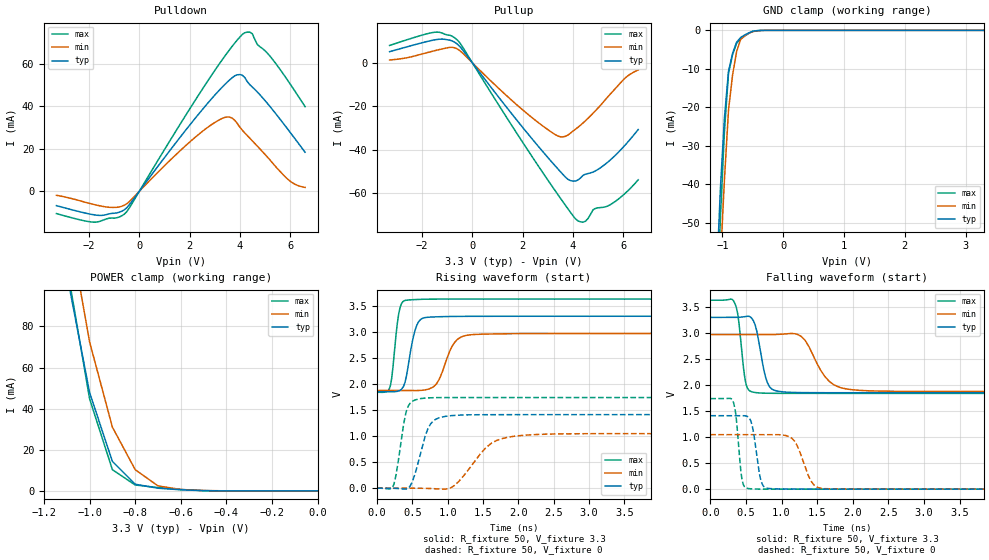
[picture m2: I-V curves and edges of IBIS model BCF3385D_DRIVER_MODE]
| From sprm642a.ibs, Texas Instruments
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|   Model Cell BCF3385D_DRIVER_MODE
|BCF3385D_DRIVER_MODE
[Model]   BCF3385D_DRIVER_MODE
Model_type   I/O
Polarity   Non-Inverting
Enable   Active-Low
Vinl =  0.8
Vinh =  2
Cref =  15.0000pF
Rref =  100.0000M
Vref =  0V
Vmeas =  1.65
C_comp   1.187844p   1.059102p   1.312744p
[Model Spec]
Vinl   0.8   0.8   0.8
Vinh   2   2   2
[Temperature Range]   25   155   -40
[Voltage Range]   3.3   2.97   3.63
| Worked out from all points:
|   slope of the pulldown table from 0 to 0.495 V, typ, clamps not added: 62.6 ohm
|   slope of the pullup table from 0 to 0.495 V, typ, clamps not added: 65.4 ohm
|   GND clamp passes 1 mA (typ) near -0.61 V on its own axis
|   POWER clamp passes 1 mA (typ) near -0.66 V on its own axis
|   rising waveform, R_fixture 50, V_fixture 3.3: 20-80 % time 120ps typ, 194ps min, 83.7ps max; typ from 1.85 V to 3.3 V
|   rising waveform, R_fixture 50, V_fixture 0: 20-80 % time 178ps typ, 387ps min, 119ps max; typ from 0 V to 1.41 V
|   falling waveform, R_fixture 50, V_fixture 3.3: 20-80 % time 122ps typ, 275ps min, 84ps max; typ from 3.3 V to 1.85 V
|   falling waveform, R_fixture 50, V_fixture 0: 20-80 % time 90.6ps typ, 176ps min, 67.2ps max; typ from 1.41 V to 0 V
| Nom Voltages:
|   VDD=1.2, VDDS=3.3, VSS=0
| Min Voltages:
|   VDD=1.08, VDDS=2.97, VSS=0
| Max Voltages:
|   VDD=1.32, VDDS=3.63, VSS=0
[POWER_clamp]
|   voltage   I(typ)   I(min)   I(max)
-3.3V     1.862A     2.383A     2.005A
-1.1V     105.5mA    134.9mA    109.6mA
-1.067V   86.28mA    114.1mA    88.01mA
-1.033V   67.04mA    93.25mA    66.38mA
-1V       47.79mA    72.42mA    44.74mA
-900mV    14.34mA    31.02mA    10.32mA
-800mV    3.256mA    10.34mA    2.892mA
-700mV    1.317mA    2.452mA    1.619mA
-600mV    561.5uA    699.2uA    696.1uA
-400mV    9.337uA    32.84uA    7.233uA
0V        61.38pA    4.167nA    15.33pA
[Pulldown]
|   voltage   I(typ)   I(min)   I(max)
-3.3V     -6.777mA   -1.903mA   -10.52mA
-1.8V     -11.11mA   -6.251mA   -14.58mA
-600mV    -8.766mA   -6.586mA   -10.8mA
1.8V      28.12mA    21.03mA    34.95mA
3.1V      46.58mA    33.11mA    58.62mA
3.7V      53.6mA     34.47mA    68.41mA
4.2V      53.63mA    27.51mA    74.77mA
4.5V      49.16mA    23.78mA    74.27mA
4.7V      46.82mA    21.27mA    69.22mA
5.2V      40.02mA    14.83mA    63.77mA
5.9V      29.45mA    5.807mA    52.45mA
6.6V      18.42mA    1.818mA    39.92mA
[Pullup]
|   voltage   I(typ)   I(min)   I(max)
-3.3V     5.214mA    1.365mA    8.091mA
-1.5V     10.67mA    5.669mA    14.19mA
-600mV    8.684mA    6.438mA    10.58mA
1.7V      -25.47mA   -18.67mA   -31.32mA
3.2V      -46.32mA   -32.39mA   -57.47mA
3.7V      -52.73mA   -33.93mA   -65.75mA
4.2V      -54.11mA   -29.76mA   -72.96mA
4.5V      -51.41mA   -26.71mA   -73.14mA
4.8V      -50.42mA   -23.27mA   -67.9mA
5.4V      -45.73mA   -15.53mA   -66.04mA
6.1V      -37.69mA   -6.785mA   -60.05mA
6.6V      -30.8mA    -3.241mA   -54.01mA
[GND_clamp]
|   voltage   I(typ)   I(min)   I(max)
-3.3V     -1.421A    -1.358A    -2.122A
-1.1V     -65.91mA   -84.58mA   -78.35mA
-1.033V   -41.08mA   -60mA      -48.65mA
-966.7mV  -22.66mA   -38.71mA   -26.25mA
-900mV    -10.66mA   -20.72mA   -11.14mA
-833.3mV  -6.012mA   -11.63mA   -6.322mA
-766.7mV  -3.075mA   -5.516mA   -3.359mA
-700mV    -1.849mA   -2.372mA   -2.258mA
-566.7mV  -654.3uA   -741.3uA   -792.3uA
-500mV    -227.6uA   -323.6uA   -256.6uA
-366.7mV  -13.17uA   -39.71uA   -12.33uA
3.3V      61.38pA    6.729uA    8.3pA
[Ramp]
| variable   typ   min   max
dV/dt_f 0.88250598/0.12344738n 0.66917746/0.27976881n  1.0870389/85.421612p
dV/dt_r 0.85760101/0.18040965n 0.64007147/0.39388755n  1.0525244/0.12019027n
R_load = 50
[Rising Waveform]
R_fixture = 50
V_fixture = 3.3
V_fixture_min = 2.97
V_fixture_max = 3.63
|   time   V(typ)   V(min)   V(max)
0s        1.852V     1.876V     1.84V
173.7ps   1.851V     1.876V     1.911V
324.6ps   1.879V     1.876V     3.467V
457.6ps   2.502V     1.874V     3.614V
535.8ps   3.026V     1.873V     3.62V
632.3ps   3.254V     1.878V     3.626V
837.5ps   3.289V     1.997V     3.629V
1.138ns   3.297V     2.858V     3.63V
1.445ns   3.299V     2.954V     3.63V
20.01ns   3.3V       2.97V      3.63V
[Rising Waveform]
R_fixture = 50
V_fixture = 0
V_fixture_min = 0
V_fixture_max = 0
|   time   V(typ)   V(min)   V(max)
0s        0V         0V         0V
237.4ps   -2.953mV   0V         76mV
400.2ps   -17.72mV   0V         1.407V
464.1ps   32.19mV    0V         1.625V
680.1ps   996.4mV    -3.954mV   1.729V
792.3ps   1.288V     -9.299mV   1.736V
954.6ps   1.375V     -19.64mV   1.739V
1.619ns   1.41V      862.3mV    1.74V
2.215ns   1.411V     1.027V     1.739V
20.03ns   1.411V     1.047V     1.74V
[Falling Waveform]
R_fixture = 50
V_fixture = 3.3
V_fixture_min = 2.97
V_fixture_max = 3.63
|   time   V(typ)   V(min)   V(max)
0s        3.3V       2.97V      3.63V
328.5ps   3.3V       2.97V      3.616V
383.8ps   3.301V     2.97V      3.38V
506.5ps   3.32V      2.97V      1.997V
689.9ps   2.767V     2.97V      1.848V
894.9ps   1.902V     2.971V     1.841V
1.234ns   1.856V     2.968V     1.841V
1.669ns   1.853V     2.073V     1.841V
2.21ns    1.853V     1.891V     1.841V
20.01ns   1.852V     1.876V     1.841V
[Falling Waveform]
R_fixture = 50
V_fixture = 0
V_fixture_min = 0
V_fixture_max = 0
|   time   V(typ)   V(min)   V(max)
0s        1.411V     1.047V     1.74V
310.5ps   1.412V     1.047V     1.714V
454ps     1.413V     1.047V     133.9mV
589.5ps   1.215V     1.047V     5.165mV
723.5ps   114.2mV    1.048V     0V
885.5ps   7.574mV    1.048V     0V
1.182ns   0V         926.9mV    0V
1.415ns   0V         154.6mV    0V
1.601ns   0V         10.09mV    0V
20.03ns   0V         0V         0V
